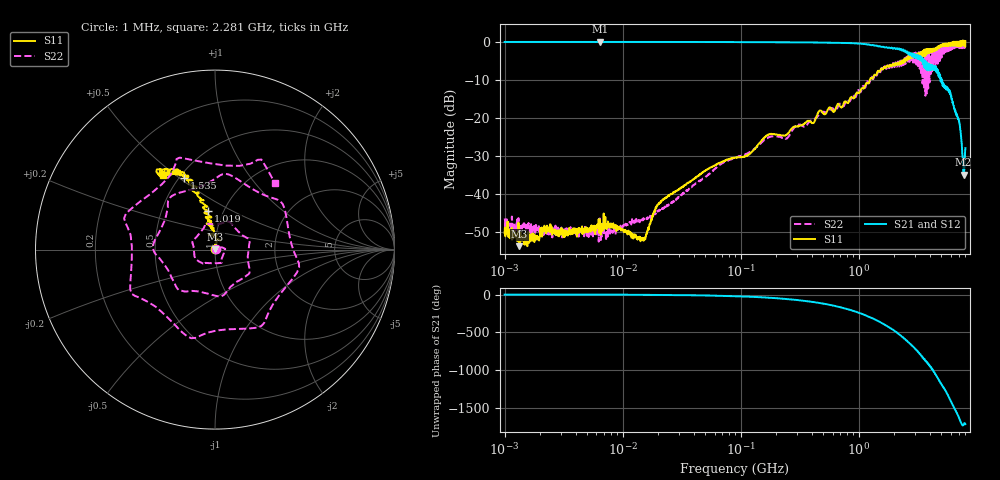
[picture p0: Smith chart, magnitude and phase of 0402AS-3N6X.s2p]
!s-Parameter Generated by FASTRON Sdn. Bhd.
!FASTRON P/N : 0402AS-3N6X
!Keysight Technologies: E5071C_MY46733604_B.14.02
!Date: Mon Dec 01 10:23:02 2025
!Version  :Rev00  Mon Dec 01 10:23:02 2025
!Data & Calibration Information:
!Freq  S11:SOLT2(ON)  S21:SOLT2(ON)  S12:SOLT2(ON)  S22:SOLT2(ON)
!PortZ  Port1:50+j0  Port2:50+j0
!When reading reference impedance value at option line is always used.
! Remarks : This data is being provided solely for informational purposes.
# Hz S dB R 50
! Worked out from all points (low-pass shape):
!   1601 points, 1 MHz to 8 GHz, reference 50 ohm
!   highest |S21| = 0.02 dB at 6.4 MHz (marker M1); lowest = -35.0 dB at 7.73 GHz (marker M2)
!   |S21| within 3 dB of the highest: start of sweep to 2.605 GHz; 2.656 GHz to 2.69 GHz (34.14 MHz wide, 1.28 % of centre)
!   lowest |S11| = -53.8 dB at 1.337 MHz (marker M3), VSWR 1.00, Z = 50.2 + j0.0694 ohm
!   |S11| at or under -10 dB: start of sweep to 1.241 GHz
!   |S22| runs from -52.6 to -0.6 dB; largest |S21 - S12| = 0.017
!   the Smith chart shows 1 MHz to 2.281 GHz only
!   S11 on the Smith chart (normalised r, x): 1 MHz: 1.01, +0.00; 1.019 GHz: 0.85, +0.38; 1.535 GHz: 0.53, +0.52; 2.281 GHz: 0.41, +0.45
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1000000  -50.30 24.6  -0.05 -0.2  -0.03 -0.3  -46.50 20.2
1336641  -53.80 19.8  -0.04 -0.4  -0.03 -0.4  -48.50 -0.1
4479405  -50.00 21.9  -0.05 -1.1  -0.02 -1.1  -49.70 30.7
6400096  -46.80 27.7  0.02 -1.5  0.07 -1.7  -46.50 11.5
2.00676e7  -42.70 30.2  -0.04 -4.9  -0.04 -4.9  -44.50 62.7
8.994653e7  -30.50 90.5  -0.07 -21.9  -0.06 -21.8  -30.50 23.5
4.006501e8  -21.40 108.0  -0.17 -96.3  -0.16 -96.3  -20.70 -126.0
7.235966e8  -17.10 95.4  -0.28 -174.0  -0.28 -174.0  -16.80 100.0
1.019114e9  -13.20 100.0  -0.48 115.0  -0.47 115.0  -13.10 -47.8
1.535164e9  -7.22 113.0  -1.26 -8.5  -1.25 -8.5  -7.69 46.7
1.7949e9  -6.66 115.0  -1.49 -68.4  -1.49 -68.4  -6.72 -73.2
2.018602e9  -5.90 123.0  -1.72 -122.0  -1.71 -122.0  -6.42 170.0
2.281485e9  -5.92 125.0  -1.89 175.0  -1.87 175.0  -6.05 47.8
2.545586e9  -4.42 129.0  -2.83 113.0  -2.80 113.0  -3.94 -83.6
2.750998e9  -4.08 131.0  -3.27 65.7  -3.22 65.6  -3.58 -179.0
2.985754e9  -3.76 143.0  -3.52 7.3  -3.49 7.1  -5.53 47.8
3.284549e9  -3.21 148.0  -4.42 -65.7  -4.39 -66.0  -7.09 -110.0
3.771001e9  -1.91 155.0  -7.39 -175.0  -7.36 -175.0  -13.60 36.4
4.216915e9  -2.63 163.0  -6.19 86.1  -6.19 85.6  -1.82 -174.0
4.548578e9  -1.54 163.0  -7.99 6.0  -8.03 5.5  -5.44 37.1
7.730116e9  0.05 -83.8  -35.00 85.0  -35.00 84.7  -0.59 -77.6
8e9  0.14 -87.8  -28.00 91.4  -28.00 91.2  -1.50 152.0
